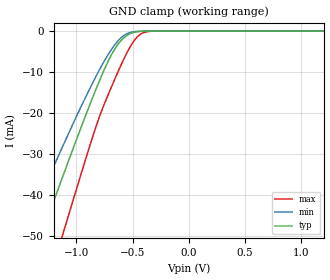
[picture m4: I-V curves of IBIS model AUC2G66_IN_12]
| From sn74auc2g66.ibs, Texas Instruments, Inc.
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[Model]   AUC2G66_IN_12
Model_type  Input
Vinl=0.385
Vinh=0.845
| variable   typ   min   max
C_comp   2.05pF   1.70pF   2.34pF
[Temperature Range]   40   100   -40
| Ambient temperature   25   85   -40
[Voltage range]   1.2   1.1   1.3
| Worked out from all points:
|   GND clamp passes 1 mA (typ) near -0.55 V on its own axis
[GND Clamp]
| AUC2G66_IN_12
|   Voltage   I(typ)   I(min)   I(max)
-2.7V     -157mA     -130.3mA   -191.7mA
-1.46V    -61.1mA    -49.11mA   -80.32mA
-1.325V   -50.8mA    -40.61mA   -68.07mA
-1.28V    -47.39mA   -37.81mA   -63.99mA
-1.12V    -35.37mA   -27.99mA   -49.46mA
-1.085V   -32.77mA   -25.89mA   -46.28mA
-745mV    -8.996mA   -6.996mA   -17.34mA
-645mV    -3.824mA   -2.884mA   -10.87mA
-545mV    -988.6uA   -575.2uA   -5.025mA
-450mV    -123.7uA   -59.61uA   -1.212mA
-350mV    -7.271uA   -4.093uA   -74.92uA
1.2V      133.3pA    224.2pA    123.7pA
